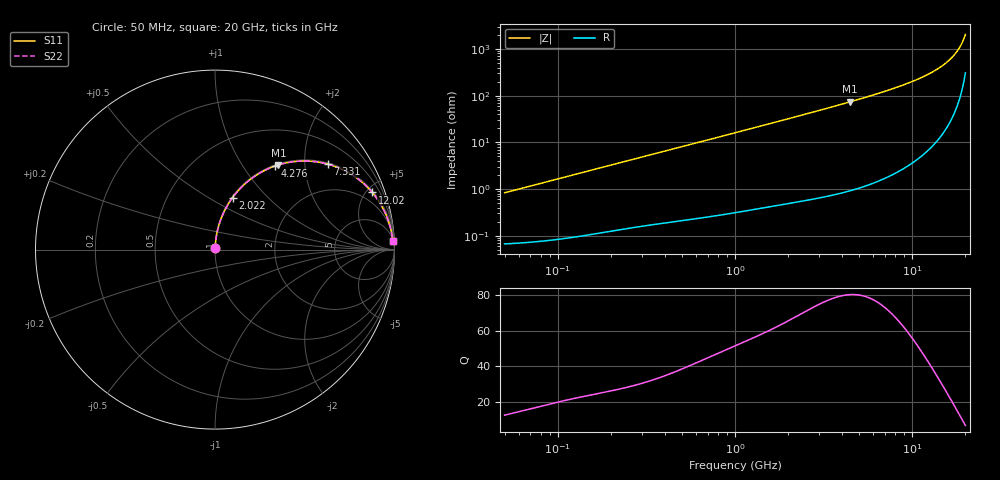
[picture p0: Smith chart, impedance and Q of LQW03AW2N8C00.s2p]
!Murata Part Number: LQW03AW2N8C00
!These Parameters are Measured in Series Mode Connection
!  o--[Z]--o
!Port1  Port2
!  o-------o
!Freq. Start=50[MHz] Stop=20[GHz], 401[Steps]
# Hz S RI R 50
!Freq.(Hz) S11(Real) S11(Imag) S21(Real) S21(Imag) S12(Real) S12(Imag) S22(Real) S22(Imag)
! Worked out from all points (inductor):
!   401 points, 50 MHz to 20 GHz, reference 50 ohm
!   read as one part in series: L = 2.63 nH near 51.52 MHz
!   highest Q = 80.5 at 4.472 GHz (marker M1), where L = 2.62 nH
!   S11 on the Smith chart (normalised r, x): 50 MHz: 1.00, +0.02; 2.022 GHz: 1.01, +0.65; 4.276 GHz: 1.02, +1.40; 7.331 GHz: 1.04, +2.61; 12.02 GHz: 1.12, +5.46; 20 GHz: 7, +40
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5e7  0.000733 0.00826  0.9993 -0.00826  0.9993 -0.00826  0.000733 0.00826
1.364002e8  0.00148 0.0223  0.9985 -0.0223  0.9985 -0.0223  0.00148 0.0223
3.721004e8  0.00536 0.0596  0.9946 -0.0596  0.9946 -0.0596  0.00536 0.0596
6.285508e8  0.0123 0.0993  0.9877 -0.0993  0.9877 -0.0993  0.0123 0.0993
1e9  0.0277 0.1548  0.9723 -0.1548  0.9723 -0.1548  0.0277 0.1548
1.476162e9  0.0559 0.2215  0.9441 -0.2215  0.9441 -0.2215  0.0559 0.2215
2.021818e9  0.0981 0.29  0.9019 -0.29  0.9019 -0.29  0.0981 0.29
2.728004e9  0.1645 0.3639  0.8355 -0.3639  0.8355 -0.3639  0.1645 0.3639
3.415248e9  0.2371 0.4189  0.7629 -0.4189  0.7629 -0.4189  0.2371 0.4189
4.275624e9  0.332 0.4648  0.668 -0.4648  0.668 -0.4648  0.332 0.4648
4.472136e9  0.3536 0.4719  0.6464 -0.4719  0.6464 -0.4719  0.3536 0.4719
5.769027e9  0.4894 0.4936  0.5106 -0.4936  0.5106 -0.4936  0.4894 0.4936
7.331367e9  0.628 0.4764  0.372 -0.4764  0.372 -0.4764  0.628 0.4764
7.442007e9  0.6367 0.474  0.3633 -0.474  0.3633 -0.474  0.6367 0.474
9.600142e9  0.7755 0.4088  0.2245 -0.4088  0.2245 -0.4088  0.7755 0.4088
1.201863e10  0.8761 0.3184  0.1239 -0.3184  0.1239 -0.3184  0.8761 0.3184
1.438523e10  0.9357 0.23  0.0643 -0.23  0.0643 -0.23  0.9357 0.23
1.550395e10  0.9544 0.1903  0.0456 -0.1903  0.0456 -0.1903  0.9544 0.1903
1.646126e10  0.9668 0.1576  0.0332 -0.1576  0.0332 -0.1576  0.9668 0.1576
1.747767e10  0.9767 0.1242  0.0233 -0.1242  0.0233 -0.1242  0.9767 0.1242
1.828096e10  0.9827 0.0989  0.0173 -0.0989  0.0173 -0.0989  0.9827 0.0989
2e10  0.9904 0.0476  0.00958 -0.0476  0.00958 -0.0476  0.9904 0.0476
